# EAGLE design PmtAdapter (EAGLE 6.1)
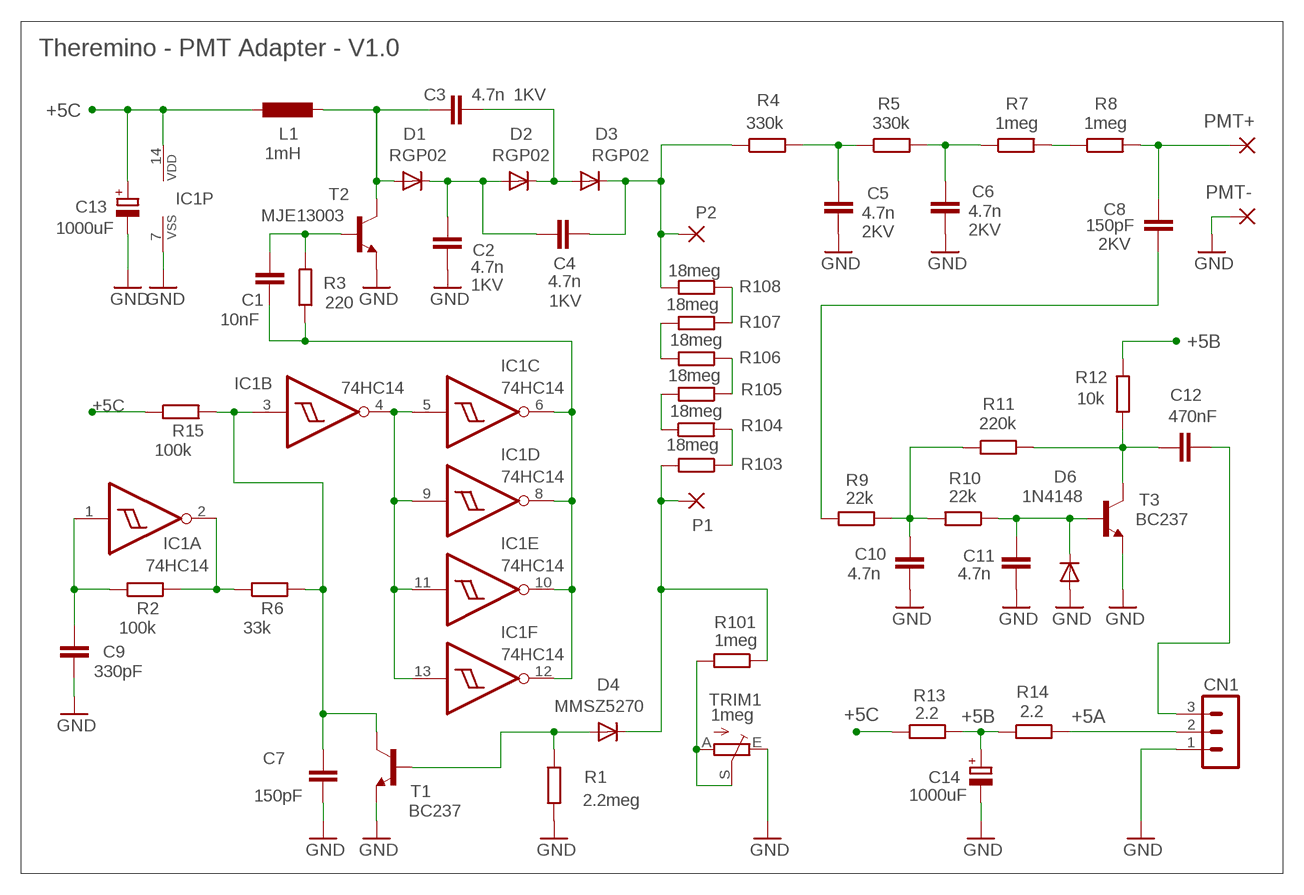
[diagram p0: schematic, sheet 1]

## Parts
C1  10nF  C-EU075-032X103  [C075-032X103]
C2  4.7n  C7.5/3  [C7.5B3]
C3  4.7n  C7.5/3  [C7.5B3]
C4  4.7n  C7.5/3  [C7.5B3]
C5  4.7n  C10/4  [C10B4]
C6  4.7n  C10/4  [C10B4]
C7  150pF  C-EU050-024X044  [C050-024X044]
C8  150pF  C7.5/3  [C7.5B3]
C9  330pF  C-EU050-024X044  [C050-024X044]
C10  4.7n  C-EU050-024X044  [C050-024X044]
C11  4.7n  C-EU050-024X044  [C050-024X044]
C12  470nF  C-EU050-024X044  [C050-024X044]
C13  1000uF  CPOL-EUE5-10.5  [E5-10,5]
C14  1000uF  CPOL-EUE5-10.5  [E5-10,5]
CN1  MA03-1N  [MA03-1]
D1  RGP02  DIODE-DO34-7  [DO34-7]
D2  RGP02  DIODE-DO34-7  [DO34-7]
D3  RGP02  DIODE-DO34-7  [DO34-7]
D4  MMSZ5270  DIODE-DO34-7  [DO34-7]
D6  1N4148  DIODE-D-5  [D-5]
IC1  74HC14  40106N  [DIL14]
L1  1mH  INDUCTORL_VERT_508  [L_VERT_508]
P1  WIREPAD1,6/0,8  [1,6/0,8]
P2  WIREPAD1,6/0,8  [1,6/0,8]
PAD1  PMT+  WIREPAD2,15/1,0  [2,15/1,0]
PAD2  PMT-  WIREPAD2,15/1,0  [2,15/1,0]
R1  2.2meg  R-EU_0207/10  [0207/10]
R2  100k  R-EU_0207/10  [0207/10]
R3  220  R-EU_0207/10  [0207/10]
R4  330k  R-EU_0207/10  [0207/10]
R5  330k  R-EU_0207/10  [0207/10]
R6  33k  R-EU_0207/10  [0207/10]
R7  1meg  R-EU_0207/10  [0207/10]
R8  1meg  R-EU_0207/10  [0207/10]
R9  22k  R-EU_0207/10  [0207/10]
R10  22k  R-EU_0207/10  [0207/10]
R11  220k  R-EU_0207/10  [0207/10]
R12  10k  R-EU_0207/10  [0207/10]
R13  2.2  R-EU_0207/10  [0207/10]
R14  2.2  R-EU_0207/10  [0207/10]
R15  100k  R-EU_0207/10  [0207/10]
R101  1meg  R-EU_0207/10  [0207/10]
R103  18meg  R-EU_R1206  [R1206]
R104  18meg  R-EU_R1206  [R1206]
R105  18meg  R-EU_R1206  [R1206]
R106  18meg  R-EU_R1206  [R1206]
R107  18meg  R-EU_R1206  [R1206]
R108  18meg  R-EU_R1206  [R1206]
T1  BC237  -NPN-TO92-CBE  [TO92-CBE]
T2  MJE13003  -NPN-TO92-BCE  [TO92-BCE]
T3  BC237  -NPN-TO92-CBE  [TO92-CBE]
TRIM1  1meg  TRIM_EU-PT10  [PT-10]

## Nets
+5A: CN1.2 R14.2
+5B: C14.+ R12.2 R13.2 R14.1
+5C: C13.+ IC1.14(P:VDD) L1.- R13.1 R15.1
GND: C2.2 C5.2 C6.2 C7.2 C9.2 C10.1 C11.1 C13.- C14.- CN1.1 D6.A IC1.7(P:VSS) PAD2.1(P) R1.2 T1.E T2.E T3.E TRIM1.E
N$1: C1.2 IC1.6(C:O) IC1.8(D:O) IC1.10(E:O) IC1.12(F:O) R3.1
N$2: IC1.4(B:O) IC1.5(C:I) IC1.9(D:I) IC1.11(E:I) IC1.13(F:I)
N$3: C12.2 R11.2 R12.1 T3.C
N$4: D4.A R1.1 T1.B
N$5: C1.1 R3.2 T2.B
N$6: C9.1 IC1.1(A:I) R2.1
N$7: IC1.2(A:O) R2.2 R6.1
N$8: C8.2 PAD1.1(P) R8.2
N$9: C2.1 C4.2 D1.C D2.A
N$10: C3.2 D2.C D3.A
N$11: R101.2 TRIM1.A TRIM1.S
N$12: C4.1 D3.C P2.1(P) R4.1 R108.2
N$13: C5.1 R4.2 R5.1
N$14: C7.1 IC1.3(B:I) R6.2 R15.2 T1.C
N$15: C6.1 R5.2 R7.1
N$16: C3.1 D1.A L1.+ T2.C
N$18: C11.2 D6.C R10.1 T3.B
N$19: C8.1 R9.2
N$24: R105.1 R106.1
N$25: R107.1 R108.1
N$26: R104.1 R105.2
N$27: R106.2 R107.2
N$28: R103.1 R104.2
N$29: D4.C P1.1(P) R101.1 R103.2
N$30: C10.2 R9.1 R10.2 R11.1
N$31: R7.2 R8.1
N$32: C12.1 CN1.3

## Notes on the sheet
- Theremino - PMT Adapter - V1.0

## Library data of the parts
C1 C7 C9-C12 = 00-LIVIO:C-EU: CAPACITOR, European symbol
C2-C4 = 00-LIVIO:C: CAPACITOR; VOLTAGE: 1KV
C5 C6 C8 = 00-LIVIO:C: CAPACITOR; VOLTAGE: 2KV
C13 C14 = 00-LIVIO:CPOL-EU: POLARIZED CAPACITOR, European symbol
CN1 = 03-con-lstb-M:MA03-1: PIN HEADER
D1-D4 D6 = 00-LIVIO:DIODE-: DIODE
IC1 = 40xx:40106: Hex SCHMITT TRIGGER
L1 = 00-LIVIO:INDUCTOR
P1 P2 PAD1 PAD2 = 00-LIVIO:WIREPAD: Wire PAD connect wire on PCB
R1-R15 R101 R103-R108 = 00-LIVIO:R-EU_: RESISTOR, European symbol
T1-T3 = 00-LIVIO:*-NPN-: NPN Transistror
TRIM1 = 00-LIVIO:TRIM_EU-: POTENTIOMETER

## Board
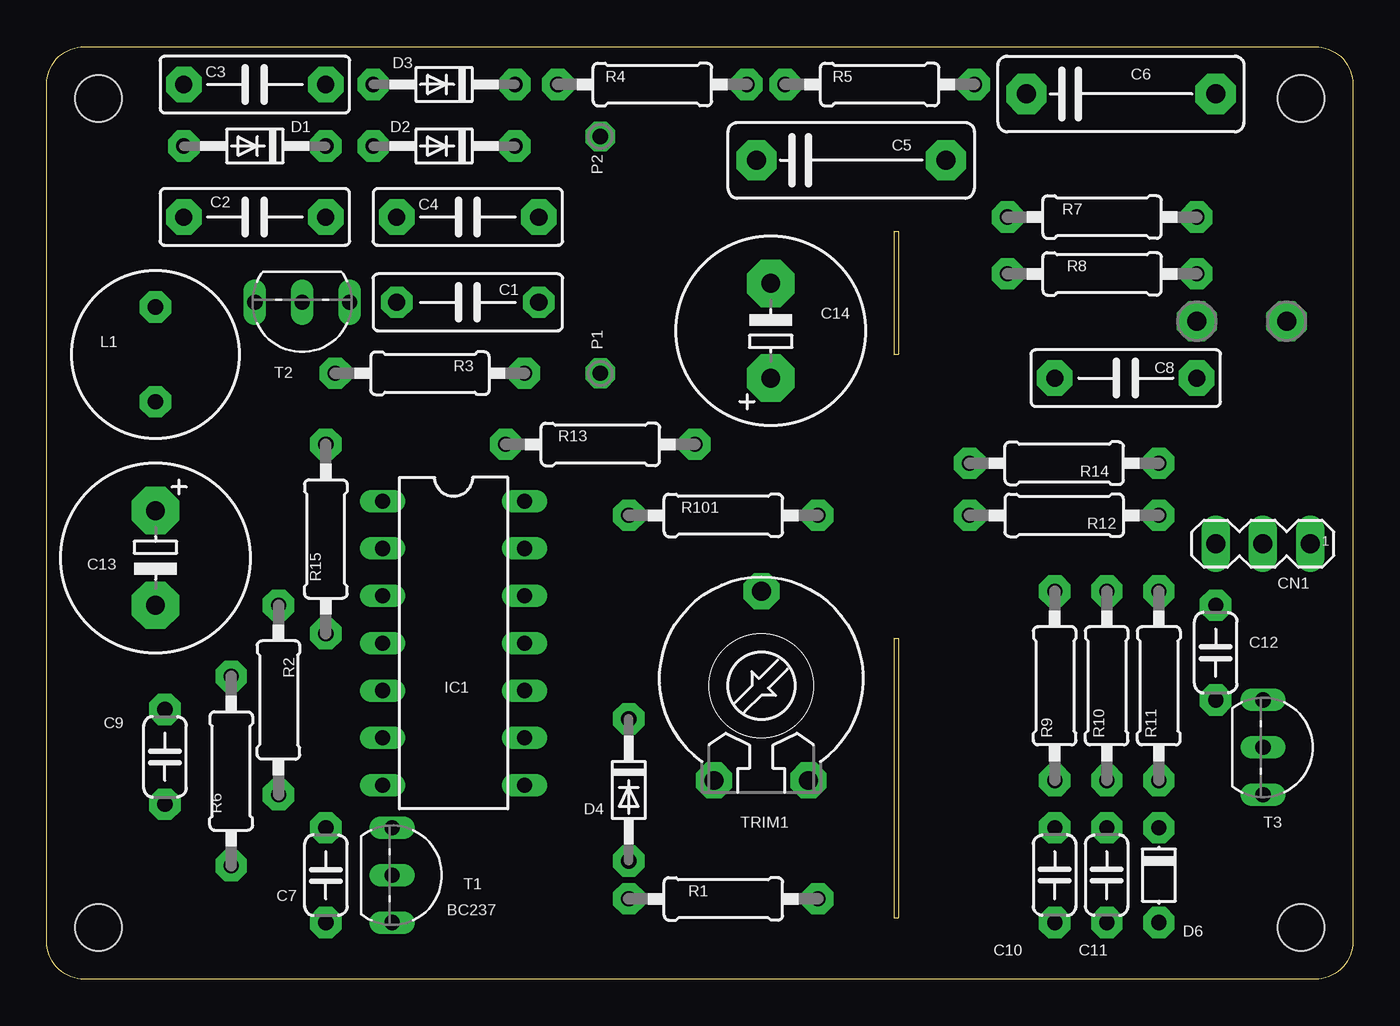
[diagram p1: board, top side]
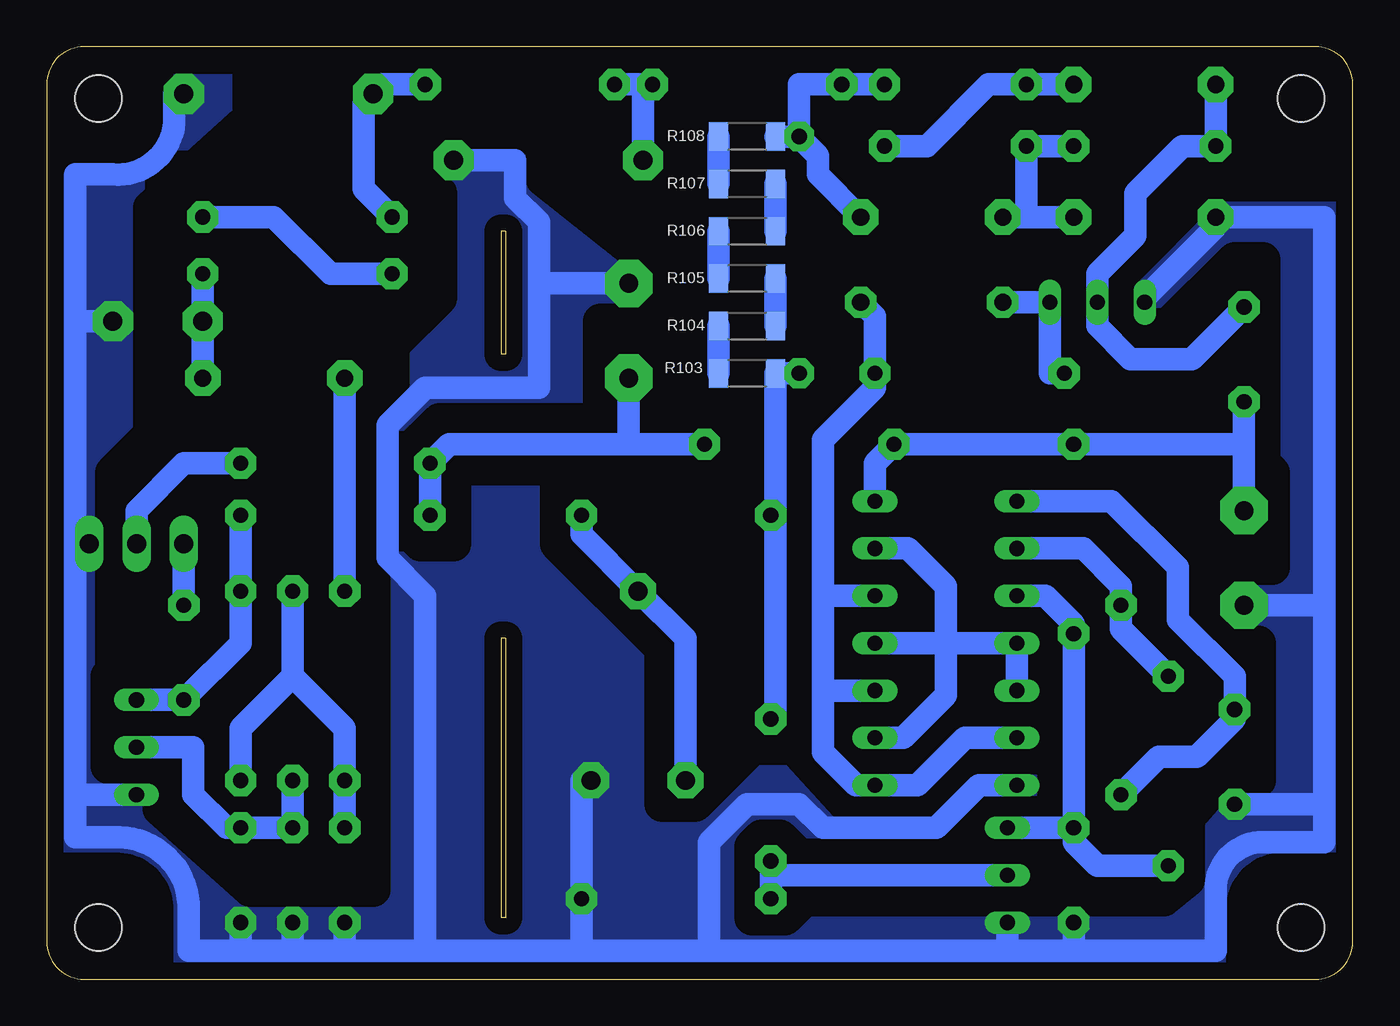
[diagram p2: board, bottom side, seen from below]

Size 70.1 x 50.04 mm. Coordinates in mm from the lower left corner, seen from the top.
Outline: 45.72,18.29 45.72,3.3
Outline: 45.72,18.29 45.72,3.3
Outline: 45.72,18.29 45.47,18.29 45.47,3.3 45.72,3.3
Outline: 2.03,0 arc-90 0,2.03 0,48.01 arc-90 2.03,50.04 68.07,50.04 arc-90 70.1,48.01 70.1,2.03 arc-90 68.07,0 2.03,0
Outline: 45.47,40.13 45.47,33.53 45.72,33.53 45.72,40.13 45.47,40.13
Copper layers (1*16): Top 0.035mm / dielectric 1.5mm / Bottom 0.035mm
Design rules: minimum track width 10mil, minimum drill 0.6mm, track to track 8mil, track to pad 8mil, pad to pad 8mil, via to via 8mil, smd to smd 8mil, copper to edge 31mil, drill to drill 8mil, minimum pad ring 5mil, minimum via ring 8mil, stop-mask expansion 4mil, vias tented up to drill 0mil, thermal gap 47mil
Holes 2.5 mm at 2.79,47.24 67.31,47.24 67.31,2.79 2.79,2.79
bRestrict: 86 lines

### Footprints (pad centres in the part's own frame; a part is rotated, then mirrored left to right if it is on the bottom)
C075-032X103 = drill 0.914 pad 1.676 octagon: 1 -3.81,0; 2 3.81,0
C7.5B3 = drill 0.914 pad 1.905 octagon: 1 -3.81,0; 2 3.81,0
C10B4 = drill 1.016 pad 2.159 octagon: 1 -5.08,0; 2 5.08,0
C050-024X044 = drill 0.813 pad 1.676 octagon: 1 -2.54,0; 2 2.54,0
E5-10,5 = drill 1.016 pad 2.54 octagon: + -2.54,0; - 2.54,0
MA03-1 = drill 1.016 long: 1 -2.54,0; 2 0,0; 3 2.54,0
DO34-7 = drill 0.813 pad 1.676 octagon: A 3.81,0; C -3.81,0
D-5 = drill 0.813 pad 1.676 octagon: A 2.54,0; C -2.54,0
DIL14 = drill 0.813 long: 1 -7.62,-3.81; 2 -5.08,-3.81; 3 -2.54,-3.81; 4 0,-3.81; 5 2.54,-3.81; 6 5.08,-3.81; 7 7.62,-3.81; 8 7.62,3.81; 9 5.08,3.81; 10 2.54,3.81; 11 0,3.81; 12 -2.54,3.81; 13 -5.08,3.81; 14 -7.62,3.81
L_VERT_508 = drill 0.813 pad 1.676 octagon: + -2.54,0; - 2.54,0
1,6/0,8 = drill 0.813 pad 1.6 octagon: 1 0,0
2,15/1,0 = drill 1.016 pad 2.159 octagon: 1 0,0
0207/10 = drill 0.813 pad 1.676 octagon: 1 -5.08,0; 2 5.08,0
R1206 = smd 1.016 x 1.524: 1 -1.524,0; 2 1.524,0
TO92-CBE = drill 0.813 long: B 0,0; C -2.54,0; E 2.54,0
TO92-BCE = drill 0.813 long: B -2.54,0; C 0,0; E 2.54,0
PT-10 = drill 1.016 pad 1.93 octagon: A -2.54,-5.08; E 2.54,-5.08; S 0,5.08

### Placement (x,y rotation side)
C1  22.61,36.32 0 top
C2  11.18,40.89 180 top
C3  11.18,48.01 0 top
C4  22.61,40.89 180 top
C5  43.18,43.94 0 top
C6  57.66,47.5 0 top
C7  14.99,5.59 270 top
C8  57.91,32.26 0 top
C9  6.35,11.94 270 top
C10  54.1,5.59 90 top
C11  56.9,5.59 90 top
C12  62.74,17.53 270 top
C13  5.84,22.61 270 top
C14  38.86,34.8 90 top
CN1  65.28,23.37 180 top
D1  11.18,44.7 180 top
D2  21.34,44.7 180 top
D3  21.34,48.01 180 top
D4  31.24,10.16 270 top
D6  59.69,5.59 270 top
IC1  21.84,18.03 270 top
L1  5.84,33.53 270 top
P1  29.72,32.51 0 top
P2  29.72,45.21 0 top
PAD1  61.72,35.31 0 top
PAD2  66.55,35.31 0 top
R1  36.32,4.32 0 top
R2  12.45,14.99 90 top
R3  20.57,32.51 180 top
R4  32.51,48.01 0 top
R5  44.7,48.01 0 top
R6  9.91,11.18 270 top
R7  56.64,40.89 0 top
R8  56.64,37.85 0 top
R9  54.1,15.75 90 top
R10  56.9,15.75 90 top
R11  59.69,15.75 90 top
R12  54.61,24.89 180 top
R13  29.72,28.7 0 top
R14  54.61,27.69 0 top
R15  14.99,23.62 270 top
R101  36.32,24.89 0 top
R103  32.51,32.51 0 bottom
R104  32.51,35.05 180 bottom
R105  32.51,37.59 0 bottom
R106  32.51,40.13 0 bottom
R107  32.51,42.67 0 bottom
R108  32.51,45.21 0 bottom
T1  18.54,5.59 270 top
T2  13.72,36.32 180 top
T3  65.28,12.45 270 top
TRIM1  38.35,15.75 0 top

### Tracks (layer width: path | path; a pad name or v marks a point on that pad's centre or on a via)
+5A
  Bottom 1.2: R14.2 62.74,27.69 65.28,25.15 CN1.2
+5B
  Bottom 1.2: R12.2 R14.1 48.51,28.7 38.86,28.7 | R13.2 38.86,28.7 | C14.+ 38.86,28.7
+5C
  Bottom 1.2: 5.84,28.7 R15.1 R13.1 25.65,27.69 IC1.14 | 5.84,28.7 C13.+ 5.84,28.7 | L1.- 5.84,28.7
GND
  Bottom 1.2: 68.58,9.91 68.58,7.62 66.55,7.62 arc90 62.48,4.06 62.48,1.52 57.4,1.52 59.69,1.52 | 68.58,9.91 68.58,17.02 68.58,23.37 | 68.58,23.37 68.58,28.96 68.58,29.46 68.58,29.97 | 68.58,29.97 68.58,35.31 | 68.58,35.31 68.58,43.18 66.55,43.18 arc-90 63.25,45.97 63.25,47.5 C6.2 | 18.54,1.52 34.54,1.52 | 34.54,1.52 41.4,1.52 | 41.4,1.52 43.69,1.52 49.78,1.52 | 1.52,20.07 1.52,24.38 | 1.52,24.38 1.52,20.07 | 1.52,20.07 1.52,9.4 | 1.52,9.4 1.52,7.37 4.83,7.37 arc-90 7.37,4.83 7.37,1.52 14.99,1.52 | 59.69,1.52 56.9,1.52 | 56.9,1.52 54.1,1.52 | 54.1,1.52 49.78,1.52 | T2.E 11.18,36.58 7.37,40.39 C2.2 1.52,40.89 1.52,24.38 | 14.99,1.52 18.54,1.52 | C13.- 1.52,20.07 | C9.2 1.52,9.4 | PAD2.1 68.58,35.31 | D6.A 59.69,1.52 | 68.58,29.72 68.58,29.97 | C11.1 56.9,1.52 | C10.1 54.1,1.52 | 49.78,1.52 49.78,20.57 51.82,22.61 51.82,29.72 49.78,31.75 43.69,31.75 43.69,37.34 | CN1.1 68.58,23.37 | TRIM1.E 41.4,10.67 R1.2 41.4,1.52 | T1.E 18.54,1.52 | C5.2 44.96,43.94 44.96,41.91 43.69,40.64 43.69,37.34 | T3.E 68.33,9.91 68.58,9.91 | IC1.7 20.07,10.41 22.35,8.13 28.45,8.13 29.72,9.4 32.51,9.4 34.54,7.37 34.54,1.52 | C7.2 14.99,1.52 | C14.- 43.69,37.34
  pour Bottom (isolate 0.9, rank 6, no thermals): -1,-1 71.1,-1 71.1,51.04 -1,51.04
N$1
  Bottom 1.2: IC1.10 28.45,15.49 | 28.45,15.49 28.45,20.57 | 28.45,20.57 IC1.12 | IC1.6 20.83,12.95 23.37,10.41 IC1.8 26.67,10.41 28.45,12.19 28.45,15.49 | 28.45,20.57 28.45,28.96 25.65,31.75 R3.1 25.65,35.56 C1.2
N$2
  Bottom 1.2: IC1.5 IC1.4 21.84,18.03 | IC1.13 23.88,23.11 21.84,21.08 21.84,18.03 | 21.84,18.03 IC1.11 | IC1.9 24.13,12.95 21.84,15.24 21.84,18.03
N$3
  Bottom 1.2: T3.C C12.2 59.69,18.03 R11.2 59.69,22.86 R12.1
N$4
  Bottom 1.2: 31.24,5.59 20.83,5.59 T1.B | R1.1 31.24,5.59 | 31.24,5.59 D4.A 31.24,5.59 | 31.24,5.59 R1.1 | R1.1 31.24,5.59
N$5
  Bottom 1.2: C1.1 T2.B 16.26,32.51 R3.2
N$6
  Bottom 1.2: 17.78,25.65 IC1.1 12.95,25.65 9.4,22.1 9.4,19.3 6.35,16.26 C9.1 6.35,13.97 8.38,11.94 10.41,11.94 R2.1
N$7
  Bottom 1.2: IC1.2 14.48,23.11 12.45,21.08 R2.2 12.45,18.8 R6.1
N$8
  Bottom 1.2: C8.2 PAD1.1 61.72,37.59 R8.2
N$9
  Bottom 1.2: D1.C D2.A 17.53,40.89 C2.1 C4.2
N$10
  Bottom 1.2: C3.2 D3.A 19.56,48.01 22.86,44.7 D2.C
N$11
  Bottom 1.2: R101.2 41.4,23.88 TRIM1.S | TRIM1.S 35.81,18.29 | TRIM1.S 35.81,18.29 | 35.81,18.29 TRIM1.A
N$12
  Bottom 1.2: R108.2 P2.1 | P2.1 29.72,48.01 R4.1 | D3.C R4.1 | C4.1 28.7,43.18 28.7,44.2 P2.1 | 28.45,48.01 R4.1
N$13
  Bottom 1.2: C5.1 38.1,48.01 | 38.1,48.01 R4.2 | R4.2 38.1,48.01 | 38.1,48.01 R5.1 38.1,48.01 | 38.1,48.01 R4.2
N$14
  Bottom 1.2: C7.1 T1.C C7.1 | C7.1 R15.2 14.99,19.05 16.51,20.57 IC1.3 | R6.2 10.16,6.1 13.72,6.1 14.99,7.37 C7.1
N$15
  Bottom 1.2: R5.2 52.07,48.01 C6.1 53.09,46.99 53.09,42.42 R7.1
N$16
  Bottom 1.2: L1.+ 8.64,33.27 11.94,33.27 13.72,35.05 T2.C 13.72,37.85 11.68,39.88 11.68,42.16 9.14,44.7 D1.A C3.1
N$18
  Bottom 1.2: T3.B 62.23,12.45 62.23,9.91 60.45,8.13 D6.C C11.2 R10.1
N$19
  Bottom 1.2: C8.1 R9.2
N$24
  Bottom 1.2: R106.1 R105.1
N$25
  Bottom 1.2: R108.1 R107.1
N$26
  Bottom 1.2: R104.1 R105.2
N$27
  Bottom 1.2: R107.2 R106.2
N$28
  Bottom 1.2: R104.2 R103.1
N$29
  Bottom 1.2: 30.99,25.15 R103.2 P1.1 | 30.99,25.15 R101.1 30.99,25.15 | 30.99,25.15 30.99,24.38 30.99,13.97 D4.C
N$30
  Bottom 1.2: C10.2 R9.1 54.1,13.46 56.9,16.26 | R11.1 59.69,13.46 56.9,16.26 | R10.2 56.9,16.26
N$31
  Bottom 1.2: R8.1 54.86,37.85 57.91,40.89 R7.2
N$32
  Bottom 1.2: CN1.3 C12.1

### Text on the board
tValues: 100 Mega | Alternative res. | Shield | Shield | Shield | Theremino - PMT Adapter - V1.0 | 50x70mm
